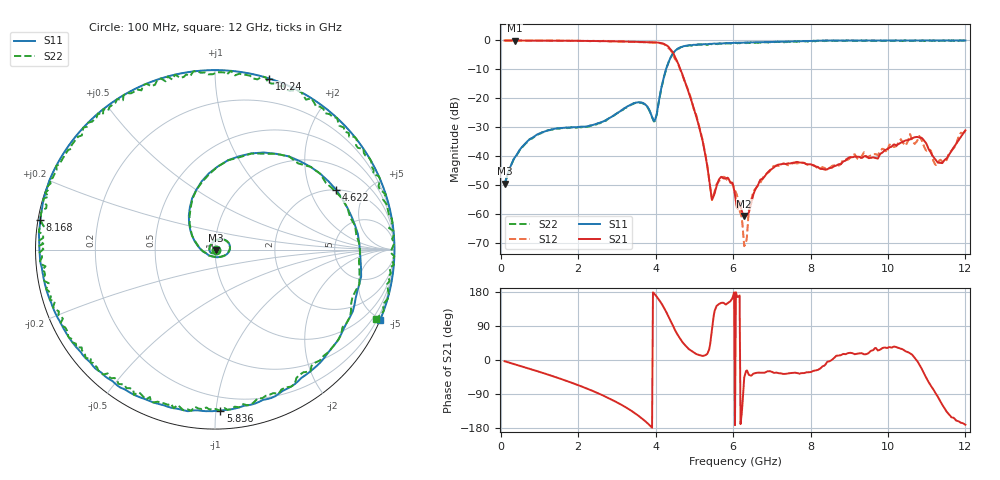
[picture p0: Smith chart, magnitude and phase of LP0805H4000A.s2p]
!	AVX	THIN	FILM	OPERATION
!	LP0805	High	Performance	Low	Pass	Filter	P/N	LP0805H4000ASTR
!	28	June	2017
#	MHz	S	dB	R	50
!	Frq	S11(dB)	S11(deg)	S21(dB)	S21(deg)	S12(dB)	S12(deg)	S22(dB)	S22(deg)
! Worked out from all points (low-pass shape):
!   501 points, 100 MHz to 12 GHz, reference 50 ohm
!   highest |S21| = -0.02 dB at 361.8 MHz (marker M1); lowest = -60.6 dB at 6.288 GHz (marker M2)
!   |S21| within 3 dB of the highest: start of sweep to 4.383 GHz
!   lowest |S11| = -49.4 dB at 100 MHz (marker M3), VSWR 1.01, Z = 50.3 - j0.154 ohm
!   |S11| at or under -10 dB: start of sweep to 4.268 GHz
!   |S22| runs from -49.6 to 0.0 dB; largest |S21 - S12| = 0.058
!   S11 on the Smith chart (normalised r, x): 100 MHz: 1.01, -0.00; 4.622 GHz: 1.99, +3.07; 5.836 GHz: 0.11, -1.03; 8.168 GHz: 0.01, +0.08; 10.24 GHz: 0.00, +1.37; 12 GHz: -0.00, -4.86
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100  -49.42 -26.9  -0.02 -3.3  0.00 -3.2  -49.62 -26.9
361.8  -40.46 -74.0  -0.02 -11.4  -0.04 -11.3  -40.46 -74.0
2099.2  -29.75 161.7  -0.15 -70.3  -0.15 -70.1  -29.95 161.5
3194  -23.39 60.6  -0.37 -122.6  -0.37 -123.0  -23.39 60.4
3955.6  -27.79 -93.9  -0.65 176.0  -0.70 174.8  -27.99 -94.1
4074.6  -21.67 177.0  -0.76 160.7  -0.84 159.7  -21.67 176.9
4336.4  -7.41 94.6  -2.26 113.9  -2.68 113.5  -7.51 94.4
4622  -2.47 26.4  -9.40 58.1  -9.60 60.6  -2.57 26.3
5121.8  -1.40 -38.0  -29.77 13.2  -29.40 12.6  -1.40 -38.2
5455  -1.18 -64.5  -55.00 81.1  -55.07 75.5  -1.28 -64.6
5835.8  -0.94 -88.1  -47.52 148.1  -47.93 151.4  -0.94 -88.2
6050  -0.79 -99.6  -53.34 -171.9  -51.78 151.8  -0.89 -99.7
6288  -0.74 -111.8  -60.63 -46.3  -71.01 173.7  -0.74 -112.0
6502.2  -0.66 -121.4  -54.39 -38.4  -53.33 -39.9  -0.86 -121.5
6835.4  -0.54 -135.9  -46.56 -32.6  -46.31 -34.4  -0.64 -136.0
8049.2  -0.14 175.2  -42.99 -29.8  -43.02 -30.3  -0.34 175.0
8168.2  -0.11 170.3  -43.61 -26.6  -43.88 -25.3  -0.11 170.2
10024.6  0.00 83.6  -37.09 33.8  -36.35 36.3  -0.20 83.4
10238.8  0.00 72.4  -36.05 33.2  -35.97 31.9  -0.20 72.4
10833.8  0.00 41.3  -33.53 -16.0  -33.49 -17.0  -0.10 41.1
11262.2  0.00 19.0  -41.73 -92.8  -42.76 -81.0  -0.10 19.0
12000  0.00 -23.2  -31.02 -170.8  -31.16 -165.0  -0.20 -23.3
